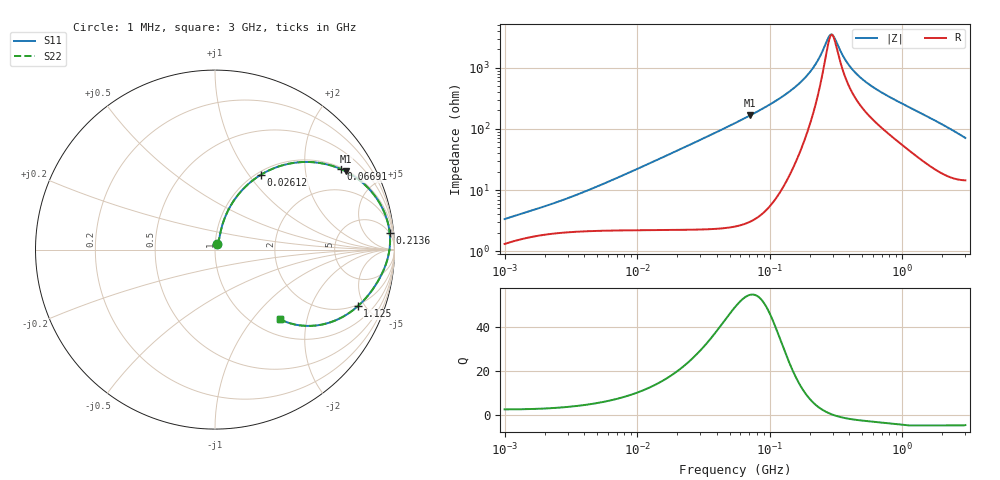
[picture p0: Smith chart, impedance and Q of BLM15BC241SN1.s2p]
! BLM15BC241SN1
# Hz S RI R 50
!Freq.(Hz) S11(Real) S11(Imag) S21(Real) S21(Imag) S12(Real) S12(Imag) S22(Real) S22(Imag)
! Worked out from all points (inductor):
!   401 points, 1 MHz to 3 GHz, reference 50 ohm
!   read as one part in series: L = 376 nH near 2.413 MHz
!   highest Q = 54.6 at 71.05 MHz (marker M1), where L = 371 nH
!   self-resonance near 296.2 MHz
!   S11 on the Smith chart (normalised r, x): 1 MHz: 1.03, +0.06; 26.12 MHz: 1.04, +1.15; 66.91 MHz: 1.06, +3.09; 213.6 MHz: 5, +20; 1.125 GHz: 1.89, -4.45; 3 GHz: 1.29, -1.39
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1000000  0.0139 0.0301  0.9861 -0.0301  0.9861 -0.0301  0.0139 0.0301
3823119  0.0278 0.0836  0.9722 -0.0836  0.9722 -0.0836  0.0278 0.0836
1.461624e7  0.1094 0.2795  0.8906 -0.2795  0.8906 -0.2795  0.1094 0.2795
2.611722e7  0.2571 0.4179  0.7429 -0.4179  0.7429 -0.4179  0.2571 0.4179
3.897472e7  0.4312 0.4821  0.5688 -0.4821  0.5688 -0.4821  0.4312 0.4821
5.477226e7  0.6048 0.4788  0.3952 -0.4788  0.3952 -0.4788  0.6048 0.4788
6.690963e7  0.702 0.4482  0.298 -0.4482  0.298 -0.4482  0.702 0.4482
7.105049e7  0.729 0.4354  0.271 -0.4354  0.271 -0.4354  0.729 0.4354
1.348146e8  0.9271 0.2417  0.0729 -0.2417  0.0729 -0.2417  0.9271 0.2417
1.714156e8  0.9595 0.1624  0.0405 -0.1624  0.0405 -0.1624  0.9595 0.1624
2.094008e8  0.9726 0.0994  0.0274 -0.0994  0.0274 -0.0994  0.9726 0.0994
2.136344e8  0.9733 0.0933  0.0267 -0.0933  0.0267 -0.0933  0.9733 0.0933
2.771263e8  0.974 0.018  0.026 -0.018  0.026 -0.018  0.974 0.018
2.942768e8  0.9722 0.00164  0.0278 -0.00164  0.0278 -0.00164  0.9722 0.00164
3.124888e8  0.9698 -0.0143  0.0302 0.0143  0.0302 0.0143  0.9698 -0.0143
3.741707e8  0.9591 -0.06  0.0409 0.06  0.0409 0.06  0.9591 -0.06
4.391493e8  0.9459 -0.0983  0.0541 0.0983  0.0541 0.0983  0.9459 -0.0983
5.696638e8  0.9181 -0.1577  0.0819 0.1577  0.0819 0.1577  0.9181 -0.1577
8.005644e8  0.8686 -0.2353  0.1314 0.2353  0.1314 0.2353  0.8686 -0.2353
1.125055e9  0.7949 -0.3159  0.2051 0.3159  0.2051 0.3159  0.7949 -0.3159
1.970482e9  0.581 -0.4203  0.419 0.4203  0.419 0.4203  0.581 -0.4203
3e9  0.3624 -0.3882  0.6376 0.3882  0.6376 0.3882  0.3624 -0.3882
